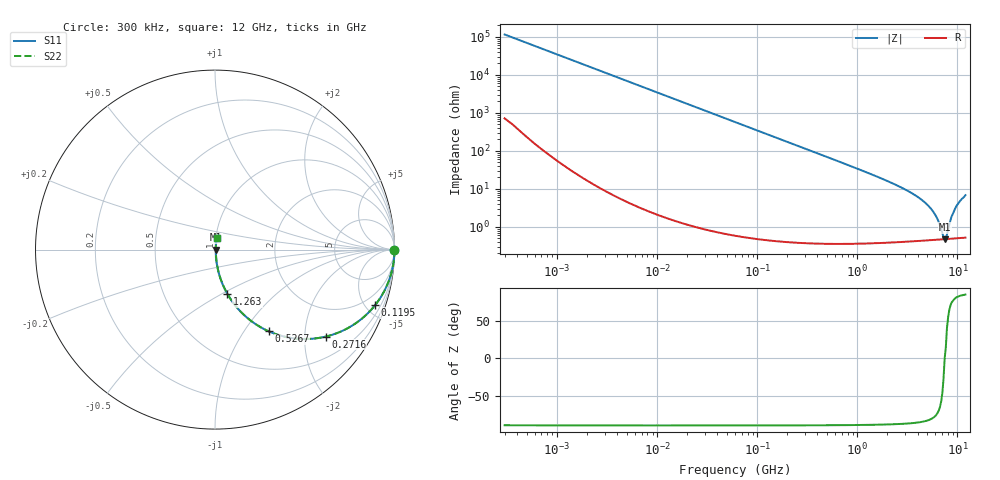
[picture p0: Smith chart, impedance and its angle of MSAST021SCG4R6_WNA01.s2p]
! MSAST021SCG4R6_WNA01  S-PARAMETER MODEL  ( General Type )
! Model Generated by TAIYO YUDEN Corporation (http://www.ty-top.com)
! Version 2.0
! TAIYO YUDEN Control No. 181101
! Copyright(c) 2015 TAIYO YUDEN CO.,LTD. All Rights Reserved.
! Product Description (link to TY-COMPAS)
! https://ds.yuden.co.jp/TYCOMPAS/or/detail?pn=MSAST021SCG4R6BWNA01&u=M
! Products Name : Multilayer Ceramic Capacitors
! Characteristics :
!  Capacitance : 4.6 pF , Rated Voltage : 25V , TCC : CG / C0G
!  Case Size : 0.25 x 0.125 / 0.0098 x 0.0049 [mm/inch] , Thickness : 0.125 / 0.0049 [mm/inch]
!  (Conditions: Temperature = 25 degC , DC Bias Current/Voltage = 0A / 0V)
! External Node Assignments :
!  1  o---| |---o  2
! GND o---------o GND
! Frequency Range : 0.3MHz  -  12000MHz  [ 401 STEP ]
# MHz S RI R 50
! Freq[MHz].  S11 Real  S11 Imag  S21 Real  S21 Imag  S12 Real  S12 Imag  S22 Real  S22 Imag
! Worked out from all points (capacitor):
!   401 points, 300 kHz to 12 GHz, reference 50 ohm
!   read as one part in series: C = 4.6 pF near 316.3 kHz
!   lowest |Z| = 475 mohm at 7.449 GHz (marker M1)
!   series resonance near 7.45 GHz, so ESL is about 99 pH
!   S11 on the Smith chart (normalised r, x): 300 kHz: open; 119.5 MHz: 1.01, -5.79; 271.6 MHz: 1.01, -2.54; 526.7 MHz: 1.01, -1.31; 1.263 GHz: 1.01, -0.53; 12 GHz: 1.01, +0.14
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0.3  1 -0.000867  6.14e-06 0.000867  6.14e-06 0.000867  1 -0.000867
1.769972  1 -0.00512  3.14e-05 0.00512  3.14e-05 0.00512  1 -0.00512
10.44266  0.9991 -0.0302  0.000928 0.0302  0.000928 0.0302  0.9991 -0.0302
60  0.9706 -0.1683  0.0294 0.1683  0.0294 0.1683  0.9706 -0.1683
119.4772  0.893 -0.3083  0.107 0.3083  0.107 0.3083  0.893 -0.3083
271.6094  0.6177 -0.4845  0.3823 0.4845  0.3823 0.4845  0.6177 -0.4845
353.9943  0.4875 -0.498  0.5125 0.498  0.5125 0.498  0.4875 -0.498
526.7124  0.3003 -0.4557  0.6997 0.4557  0.6997 0.4557  0.3003 -0.4557
804.7407  0.155 -0.3578  0.845 0.3578  0.845 0.3578  0.155 -0.3578
1262.535  0.0691 -0.2469  0.9309 0.2469  0.9309 0.2469  0.0691 -0.2469
2088.533  0.0264 -0.148  0.9736 0.148  0.9736 0.148  0.0264 -0.148
3547.679  0.00973 -0.0744  0.9903 0.0744  0.9903 0.0744  0.00973 -0.0744
5006.236  0.00581 -0.0375  0.9942 0.0375  0.9942 0.0375  0.00581 -0.0375
6026.253  0.00493 -0.0197  0.9951 0.0197  0.9951 0.0197  0.00493 -0.0197
6524.734  0.00476 -0.0122  0.9952 0.0122  0.9952 0.0122  0.00476 -0.0122
7064.448  0.0047 -0.00489  0.9953 0.00489  0.9953 0.00489  0.0047 -0.00489
7448.838  0.00473 -5.13e-06  0.9953 5.13e-06  0.9953 5.13e-06  0.00473 -5.13e-06
7854.144  0.00479 0.00407  0.9952 -0.00407  0.9952 -0.00407  0.00479 0.00407
8732.115  0.00519 0.0179  0.9948 -0.0179  0.9948 -0.0179  0.00519 0.0179
9454.42  0.0058 0.0292  0.9942 -0.0292  0.9942 -0.0292  0.0058 0.0292
10511.28  0.00714 0.0456  0.9929 -0.0456  0.9929 -0.0456  0.00714 0.0456
12000  0.00973 0.0671  0.9903 -0.0671  0.9903 -0.0671  0.00973 0.0671
